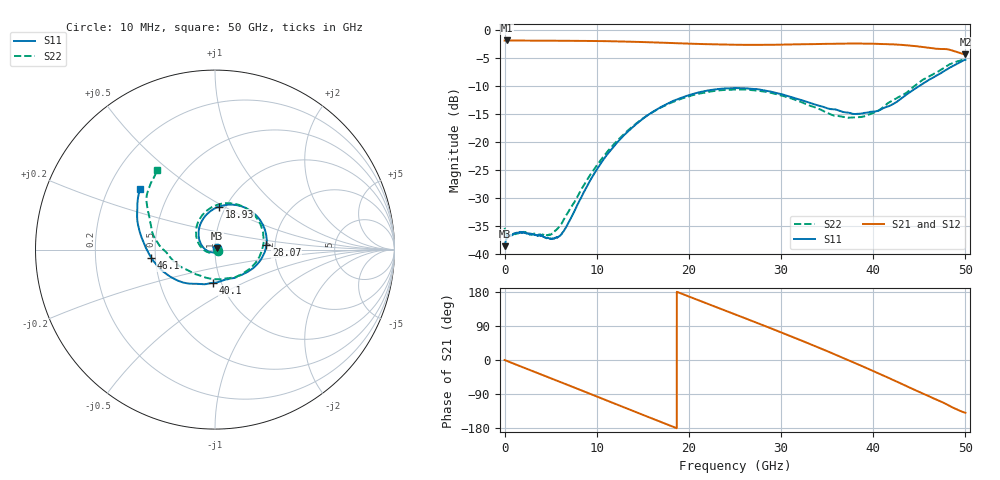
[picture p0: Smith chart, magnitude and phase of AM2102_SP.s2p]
!Keysight Technologies,N5245B,MY58422270,A.16.20.02
!Date: Wednesday, March 11, 2026 23:07:34
!Correction: S11(C  2-Port  )
!S21(C  2-Port  )
!S12(C  2-Port  )
!S22(C  2-Port  )
!S2P File: Measurements: S11, S21, S12, S22:
# Hz S  dB  R 50
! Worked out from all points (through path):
!   6401 points, 10 MHz to 50 GHz, reference 50 ohm
!   highest |S21| = -1.95 dB at 283.4 MHz (marker M1); lowest = -4.4 dB at 50 GHz (marker M2)
!   group delay of S21, straight-line fit = 27.4 ps
!   lowest |S11| = -38.7 dB at 10 MHz (marker M3), VSWR 1.02, Z = 50.9 + j0.72 ohm
!   |S11| at or under -10 dB: start of sweep to 45.06 GHz
!   |S22| runs from -37.3 to -5.2 dB; largest |S21 - S12| = 0.0067
!   S11 on the Smith chart (normalised r, x): 10 MHz: 1.02, +0.01; 18.93 GHz: 0.93, +0.48; 28.07 GHz: 1.80, +0.10; 40.1 GHz: 0.92, -0.35; 46.1 GHz: 0.47, -0.05; 50 GHz: 0.34, +0.32
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1e7  -38.68 37.4  -1.96 -0.1  -1.92 -0.5  -35.41 -22.4
2.833828e8  -36.78 1.4  -1.95 -2.8  -1.95 -2.8  -37.31 -1.2
2.970345e9  -36.55 -18.5  -1.98 -28.5  -1.98 -28.6  -36.58 -25.8
4.84497e9  -37.28 -54.4  -1.99 -46.5  -1.99 -46.5  -36.64 -67.0
5.84477e9  -37.03 -86.3  -2.00 -56.1  -2.00 -56.1  -35.37 -98.2
8.34427e9  -29.90 -156.4  -2.02 -80.2  -2.02 -80.2  -28.52 -154.0
1.218725e10  -20.23 151.1  -2.11 -117.4  -2.11 -117.4  -19.91 157.7
1.448367e10  -16.62 126.8  -2.20 -139.6  -2.21 -139.6  -16.52 135.0
1.667854e10  -14.10 105.2  -2.32 -160.7  -2.32 -160.7  -14.17 114.3
1.892809e10  -12.35 84.0  -2.46 177.7  -2.46 177.7  -12.51 94.2
2.17947e10  -10.97 58.3  -2.60 150.6  -2.60 150.7  -11.24 69.6
2.5005e10  -10.45 30.6  -2.71 120.5  -2.71 120.5  -10.71 42.3
2.80747e10  -10.85 5.2  -2.73 91.5  -2.74 91.5  -11.06 15.3
3.067574e10  -11.84 -15.4  -2.67 66.6  -2.68 66.5  -12.08 -10.3
3.333927e10  -13.21 -34.9  -2.61 40.2  -2.60 40.2  -13.71 -39.2
3.682295e10  -14.75 -61.2  -2.51 4.7  -2.51 4.7  -15.61 -87.2
4.010354e10  -14.65 -93.0  -2.54 -30.3  -2.54 -30.3  -14.80 -136.5
4.167354e10  -13.68 -112.0  -2.62 -47.2  -2.62 -47.2  -13.06 -156.9
4.387622e10  -11.30 -141.2  -2.85 -71.9  -2.85 -71.9  -10.95 -179.2
4.610234e10  -8.92 -172.6  -3.25 -96.3  -3.24 -96.3  -8.36 159.2
4.852373e10  -6.60 158.0  -3.73 -124.2  -3.71 -124.2  -6.06 138.3
5e10  -5.40 140.9  -4.44 -139.2  -4.47 -139.2  -5.19 126.1
